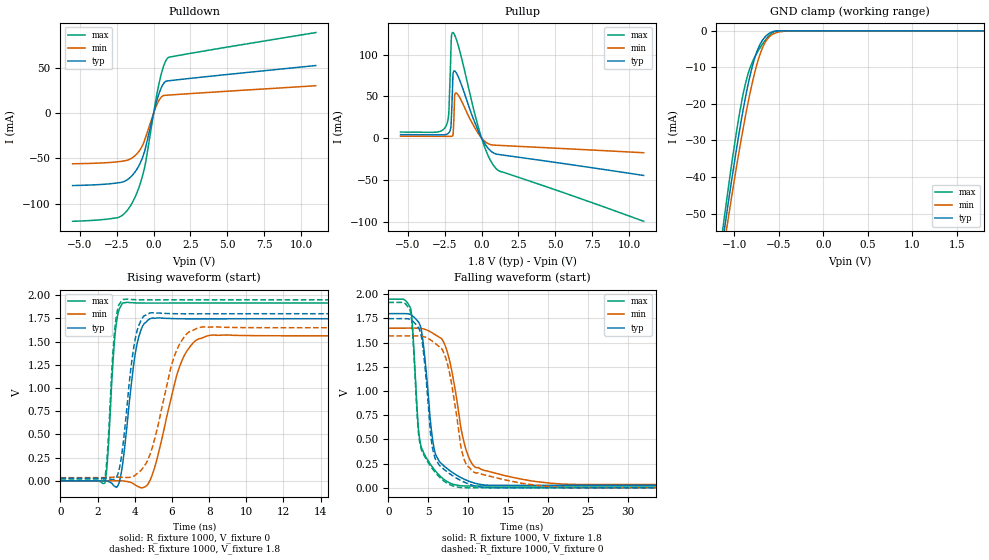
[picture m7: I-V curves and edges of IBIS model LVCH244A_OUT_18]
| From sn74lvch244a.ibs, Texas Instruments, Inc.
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[Model]   LVCH244A_OUT_18
Model_type  3-state
Enable   Active-Low
Vref =   0
Rref =   1000
Cref =   30p
Vmeas =   0.9
| variable   typ   min   max
C_comp   5.16pF   5.00pF   5.68pF
| C_pullup   6.72pF   5.79pF   7.26pF
| C_pulldown   6.56pF   4.99pF   7.66pF
| C_tri-state   5.16pF   5.00pF   5.68pF
[Temperature Range]   40   100   -40
| Ambient temperature   25   85   -40
[Voltage range]   1.8   1.65   1.95
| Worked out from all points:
|   slope of the pulldown table from 0 to 0.27 V, typ, clamps not added: 16.1 ohm
|   slope of the pullup table from 0 to 0.27 V, typ, clamps not added: 33.2 ohm
|   GND clamp passes 1 mA (typ) near -0.62 V on its own axis
|   rising waveform, R_fixture 1000, V_fixture 0: 20-80 % time 599ps typ, 1.16ns min, 336ps max; typ from 0 V to 1.75 V
|   falling waveform, R_fixture 1000, V_fixture 1.8: 20-80 % time 1.36ns typ, 2.25ns min, 1.09ns max; typ from 1.8 V to 0.026 V
|   rising waveform, R_fixture 1000, V_fixture 1.8: 20-80 % time 591ps typ, 1.17ns min, 331ps max; typ from 0.025 V to 1.8 V
|   falling waveform, R_fixture 1000, V_fixture 0: 20-80 % time 1.3ns typ, 1.94ns min, 1.1ns max; typ from 1.75 V to 0 V
[GND Clamp]
| LVCH244A_OUT_18
|   Voltage   I(typ)   I(min)   I(max)
-5.5V     -943.7mA   -897.4mA   -1.02A
-1.135V   -58.81mA   -62.42mA   -55.76mA
-1.11V    -54.52mA   -58.37mA   -51.12mA
-1.085V   -50.3mA    -54.37mA   -46.56mA
-1.06V    -46.14mA   -50.42mA   -42.09mA
-955mV    -29.59mA   -34.57mA   -24.85mA
-860mV    -16.65mA   -21.68mA   -13.21mA
-730mV    -4.808mA   -7.973mA   -5.473mA
-660mV    -1.867mA   -3.508mA   -2.857mA
-585mV    -404.1uA   -1.227mA   -780.1uA
-330mV    -956.1nA   -18.75uA   -196nA
1.8V      1.143nA    69.62nA    -1.245nA
[Pulldown]
| LVCH244A_OUT_18
|   Voltage   I(typ)   I(min)   I(max)
-5.5V     -79.87mA   -55.87mA   -119.3mA
-2.425V   -76.89mA   -53.63mA   -115.2mA
-1.965V   -75.1mA    -52.58mA   -110.4mA
-1.51V    -69.66mA   -49.87mA   -100.5mA
-1.04V    -59.11mA   -43.01mA   -83.9mA
-660mV    -44.48mA   -31.93mA   -63.05mA
-520mV    -36.04mA   -25.44mA   -52.06mA
75mV      5.11mA     3.526mA    7.487mA
360mV     21.36mA    14.01mA    32.24mA
680mV     32.74mA    19.42mA    52.05mA
980mV     35.61mA    19.85mA    61.16mA
11V       52.47mA    30.19mA    88.83mA
[Pullup]
| LVCH244A_OUT_18
|   Voltage   I(typ)   I(min)   I(max)
-5.5V     4.132mA    2.28mA     7.221mA
-2.42V    4.318mA    2.093mA    14.19mA
-2.225V   6.276mA    2.078mA    30.14mA
-2.085V   12.97mA    2.077mA    101.8mA
-2.045V   25.72mA    2.109mA    121.9mA
-1.945V   74.01mA    3.628mA    126.3mA
-1.895V   79.92mA    16.6mA     125.6mA
-1.83V    80.38mA    50.38mA    123.6mA
-1.73V    78.5mA     54.06mA    119.2mA
-25mV     874.8uA    531.1uA    1.42mA
995mV     -19.19mA   -8.546mA   -36.64mA
11V       -44.72mA   -17.52mA   -99.6mA
[Ramp]
| LVCH244A_OUT_18
| variable   typ   min   max
dV/dt_r   1.09/6.48E-10   0.99/1.28E-09   1.17/3.52E-10
dV/dt_f   1.06/1.43E-09   0.97/2.39E-09   1.16/1.14E-09
R_load = 1000
[Rising Waveform]
| LVCH244A_OUT_18
R_fixture =   1000
C_fixture =   0
L_fixture =   0
V_fixture =   0
V_fixture_min = 0
V_fixture_max = 0
|   Time   V(typ)   V(min)   V(max)
0s        658.2pV    3.504nV    29.11nV
2.39ns    -368.9uV   -468.7uV   -24.11mV
2.545ns   -5.182mV   -557.5uV   264.7mV
2.95ns    -63.89mV   481.1uV    1.597V
3.4ns     264.7mV    -2.557mV   1.918V
4.105ns   1.457V     -55.51mV   1.916V
4.91ns    1.752V     48.43mV    1.914V
6.52ns    1.745V     1.287V     1.915V
8.04ns    1.745V     1.567V     1.915V
50ns      1.746V     1.563V     1.915V
[Falling Waveform]
| LVCH244A_OUT_18
R_fixture =   1000
C_fixture =   0
L_fixture =   0
V_fixture =   1.8
V_fixture_min = 1.65
V_fixture_max = 1.95
|   Time   V(typ)   V(min)   V(max)
0s        1.8V       1.65V      1.95V
2.81ns    1.789V     1.651V     1.845V
3.945ns   1.685V     1.648V     496.2mV
4.465ns   1.425V     1.641V     353.4mV
5.74ns    401.8mV    1.589V     190.5mV
7.72ns    176.4mV    1.296V     49.06mV
9.475ns   89.92mV    471.4mV    19.32mV
10.97ns   44.81mV    209.7mV    19.17mV
21.81ns   25.64mV    38.54mV    19.05mV
50ns      25.52mV    33.68mV    18.99mV
[Rising Waveform]
| LVCH244A_OUT_18
R_fixture =   1000
C_fixture =   0
L_fixture =   0
V_fixture =   1.8
V_fixture_min = 1.65
V_fixture_max = 1.95
|   Time   V(typ)   V(min)   V(max)
0s        25.49mV    33.57mV    18.98mV
2.385ns   28.49mV    35.02mV    32.53mV
2.535ns   25.59mV    36.24mV    329.6mV
2.93ns    21.52mV    38.56mV    1.65V
3.385ns   422mV      37.6mV     1.955V
3.93ns    1.419V     48.69mV    1.952V
4.395ns   1.751V     126.4mV    1.95V
6.25ns    1.8V       1.405V     1.95V
7.57ns    1.799V     1.656V     1.95V
50ns      1.8V       1.65V      1.95V
[Falling Waveform]
| LVCH244A_OUT_18
R_fixture =   1000
C_fixture =   0
L_fixture =   0
V_fixture =   0
V_fixture_min = 0
V_fixture_max = 0
|   Time   V(typ)   V(min)   V(max)
0s        1.748V     1.57V      1.916V
2.81ns    1.737V     1.57V      1.806V
3.9ns     1.632V     1.569V     483.8mV
4.44ns    1.367V     1.562V     338mV
5.59ns    387.5mV    1.51V      189mV
6.835ns   200.1mV    1.415V     77.69mV
7.75ns    141.3mV    1.151V     29.85mV
9.305ns   66.35mV    347.8mV    1.009mV
10.87ns   18.95mV    155.5mV    209.9uV
50ns      29.1uV     101.3uV    10.59uV
